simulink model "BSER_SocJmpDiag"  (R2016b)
settings: Solver=FixedStepDiscrete  StartTime=0.0  StopTime=10.0  FixedStep=0.02  RelTol=1e-3  EnableMultiTasking=on
undefined symbols (not defined in the file or in its folder): BSER_bSocJmpDiagSlct_CW, BSER_rBattSocValJmpFault_C, BSER_tiBattSocValJmpDiag_C, BSER_tiBattSocValJmpFault_C, BSER_tiSocValJmpErr_C, BSER_tiSocValJmpOk_C
libraries: simulink x6

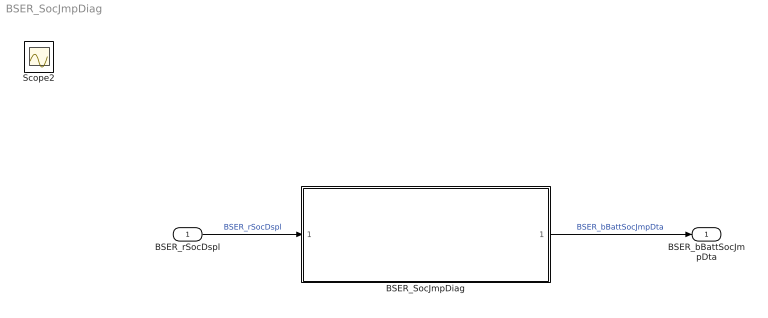
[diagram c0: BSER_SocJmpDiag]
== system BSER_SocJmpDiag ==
  BSER_rSocDspl : Inport
  BSER_SocJmpDiag : Subsystem
  BSER_bBattSocJmpDta : Outport
  Scope2 : Scope
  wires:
  BSER_rSocDspl/1 -> BSER_SocJmpDiag/1(BSER_rSocDspl)  "BSER_rSocDspl"
  BSER_SocJmpDiag/1(BSER_bBattSocJmpDta) -> BSER_bBattSocJmpDta/1  "BSER_bBattSocJmpDta"

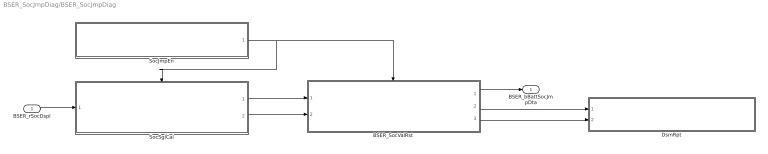
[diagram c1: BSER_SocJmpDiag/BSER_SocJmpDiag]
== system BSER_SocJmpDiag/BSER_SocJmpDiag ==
  BSER_rSocDspl : Inport
  BSER_SocValRst : Subsystem
  DsmRpt : Subsystem
  SocJmpEn : Subsystem
  SocSglCal : Subsystem
  BSER_bBattSocJmpDta : Outport
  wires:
  BSER_SocValRst/1(BSER_bBattSocJmpDta) -> BSER_bBattSocJmpDta/1
  SocJmpEn/1(BSER_bBattSocJmpEn) -> BSER_SocValRst/Enable, SocSglCal/Enable
  BSER_rSocDspl/1 -> SocSglCal/1(BSER_rSocDspl)
  SocSglCal/1(BSER_rSocDsplCont) -> BSER_SocValRst/1(BSER_rSocDsplCont)
  SocSglCal/2(BSER_rSocDsplPer) -> BSER_SocValRst/2(BSER_rSocDsplPer)
  BSER_SocValRst/2(BSER_bBattSocJmpFaultDet) -> DsmRpt/1(BSER_bBattSocJmpFaultDet)
  BSER_SocValRst/3(BSER_bBattSocJmpFaultHeal) -> DsmRpt/2(BSER_bBattSocJmpFaultHeal)

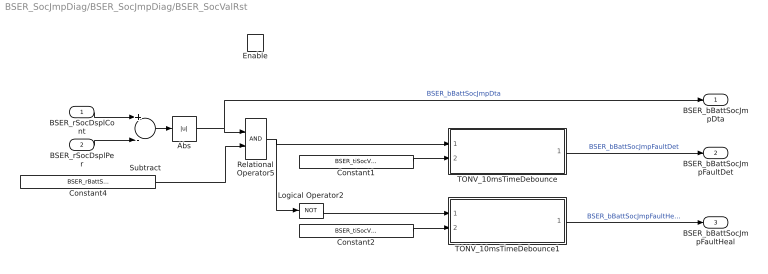
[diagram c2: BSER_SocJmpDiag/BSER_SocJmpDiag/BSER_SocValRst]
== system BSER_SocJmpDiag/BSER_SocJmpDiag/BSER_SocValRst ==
  BSER_rSocDsplCont : Inport
  BSER_rSocDsplPer : Inport  Port=2
  Enable : EnablePort  StatesWhenEnabling=reset
  Abs : Abs
  Constant1 : Constant  Value=BSER_tiSocValJmpErr_C
  Constant2 : Constant  Value=BSER_tiSocValJmpOk_C
  Constant4 : Constant  Value=BSER_rBattSocValJmpFault_C
  Logical Operator2 : Logic  Operator=NOT  AllPortsSameDT=off  OutDataTypeStr=boolean
  Relational Operator5 : RelationalOperator  OutDataTypeStr=boolean  RndMeth=Simplest
  Subtract : Sum  Inputs=+-  OutDataTypeStr=single
  TONV_10msTimeDebounce : Subsystem  TreatAsAtomicUnit=on  RTWFcnName=TONV_10msTimeDebounce  RTWFileName=SrvLib
  TONV_10msTimeDebounce1 : Subsystem  TreatAsAtomicUnit=on  RTWFcnName=TONV_10msTimeDebounce  RTWFileName=SrvLib
  BSER_bBattSocJmpDta : Outport  InitialOutput=[0]
  BSER_bBattSocJmpFaultDet : Outport  Port=2  InitialOutput=[0]
  BSER_bBattSocJmpFaultHeal : Outport  Port=3  InitialOutput=[0]
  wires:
  BSER_rSocDsplCont/1 -> Subtract/1
  Constant2/1 -> TONV_10msTimeDebounce1/2(T)
  Logical Operator2/1 -> TONV_10msTimeDebounce1/1(u)
  TONV_10msTimeDebounce1/1(y) -> BSER_bBattSocJmpFaultHeal/1  "BSER_bBattSocJmpFaultHeal"
  Constant1/1 -> TONV_10msTimeDebounce/2(T)
  TONV_10msTimeDebounce/1(y) -> BSER_bBattSocJmpFaultDet/1  "BSER_bBattSocJmpFaultDet"
  Constant4/1 -> Relational Operator5/2
  Subtract/1 -> Abs/1
  Abs/1 -> Relational Operator5/1, BSER_bBattSocJmpDta/1  "BSER_bBattSocJmpDta"
  Relational Operator5/1 -> Logical Operator2/1, TONV_10msTimeDebounce/1(u)
  BSER_rSocDsplPer/1 -> Subtract/2

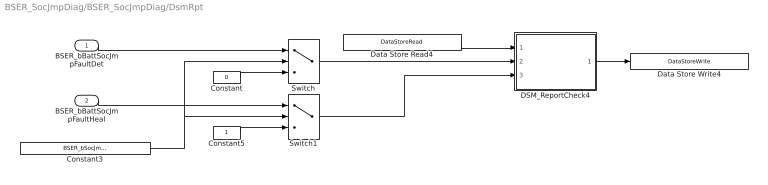
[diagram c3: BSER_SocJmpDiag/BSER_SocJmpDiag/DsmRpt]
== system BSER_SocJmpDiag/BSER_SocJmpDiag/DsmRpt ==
  BSER_bBattSocJmpFaultDet : Inport
  BSER_bBattSocJmpFaultHeal : Inport  Port=2
  Constant : Constant  Value=0  OutDataTypeStr=boolean
  Constant3 : Constant  Value=BSER_bSocJmpDiagSlct_CW
  Constant5 : Constant  OutDataTypeStr=boolean
  DSM_ReportCheck4 : Subsystem  TreatAsAtomicUnit=on  RTWFcnName=DSM_ReportCheck  RTWFileName=SrvLib
  Data Store Read4 : DataStoreRead  DataStoreName=DFC_SocValJmp
  Data Store Write4 : DataStoreWrite  DataStoreName=DFC_SocValJmp
  Switch : Switch  Criteria=u2 > Threshold
  Switch1 : Switch  Criteria=u2 > Threshold
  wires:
  DSM_ReportCheck4/1(Dfc_id) -> Data Store Write4/1
  Data Store Read4/1 -> DSM_ReportCheck4/1(Dfc_id_nv)
  Switch1/1 -> DSM_ReportCheck4/3(Heal)
  BSER_bBattSocJmpFaultDet/1 -> Switch/1
  BSER_bBattSocJmpFaultHeal/1 -> Switch1/1
  Constant/1 -> Switch/3
  Constant5/1 -> Switch1/3
  Constant3/1 -> Switch1/2, Switch/2
  Switch/1 -> DSM_ReportCheck4/2(Err)

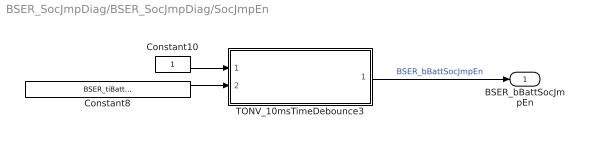
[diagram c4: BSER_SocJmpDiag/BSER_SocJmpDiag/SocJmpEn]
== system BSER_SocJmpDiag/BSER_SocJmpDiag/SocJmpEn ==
  Constant10 : Constant  OutDataTypeStr=boolean
  Constant8 : Constant  Value=BSER_tiBattSocValJmpDiag_C
  TONV_10msTimeDebounce3 : Subsystem  TreatAsAtomicUnit=on  RTWFcnName=TONV_10msTimeDebounce  RTWFileName=SrvLib
  BSER_bBattSocJmpEn : Outport
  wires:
  Constant8/1 -> TONV_10msTimeDebounce3/2(T)
  Constant10/1 -> TONV_10msTimeDebounce3/1(u)
  TONV_10msTimeDebounce3/1(y) -> BSER_bBattSocJmpEn/1  "BSER_bBattSocJmpEn"

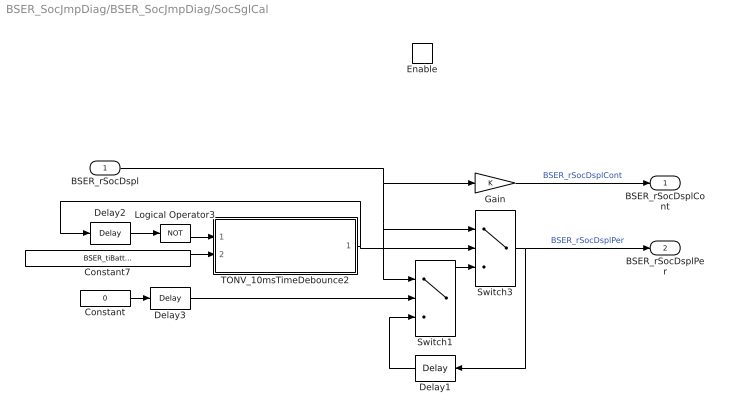
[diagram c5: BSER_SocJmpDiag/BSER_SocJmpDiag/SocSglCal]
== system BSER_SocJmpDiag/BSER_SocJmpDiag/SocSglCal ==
  BSER_rSocDspl : Inport
  Enable : EnablePort  StatesWhenEnabling=reset
  Constant : Constant  Value=0  OutDataTypeStr=uint8
  Constant7 : Constant  Value=BSER_tiBattSocValJmpFault_C
  Delay1 : Delay  DelayLength=1  InitialCondition=1
  Delay2 : Delay  DelayLength=1  InitialCondition=1
  Delay3 : Delay  DelayLength=1  InitialCondition=1
  Gain : Gain
  Logical Operator3 : Logic  Operator=NOT  AllPortsSameDT=off  OutDataTypeStr=boolean
  Switch1 : Switch  Criteria=u2 > Threshold
  Switch3 : Switch  Criteria=u2 > Threshold
  TONV_10msTimeDebounce2 : Subsystem  TreatAsAtomicUnit=on  RTWFcnName=TONV_10msTimeDebounce  RTWFileName=SrvLib
  BSER_rSocDsplCont : Outport
  BSER_rSocDsplPer : Outport  Port=2
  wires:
  Constant7/1 -> TONV_10msTimeDebounce2/2(T)
  Delay2/1 -> Logical Operator3/1
  Logical Operator3/1 -> TONV_10msTimeDebounce2/1(u)
  TONV_10msTimeDebounce2/1(y) -> Switch3/2, Delay2/1
  BSER_rSocDspl/1 -> Switch1/1, Switch3/1, Gain/1
  Switch3/1 -> BSER_rSocDsplPer/1, Delay1/1  "BSER_rSocDsplPer"
  Gain/1 -> BSER_rSocDsplCont/1  "BSER_rSocDsplCont"
  Constant/1 -> Delay3/1
  Delay3/1 -> Switch1/2
  Delay1/1 -> Switch1/3
  Switch1/1 -> Switch3/3

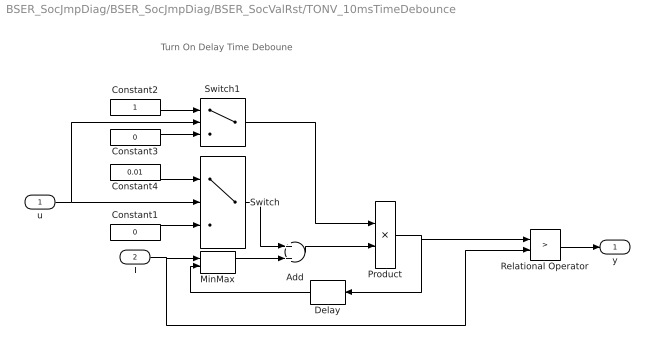
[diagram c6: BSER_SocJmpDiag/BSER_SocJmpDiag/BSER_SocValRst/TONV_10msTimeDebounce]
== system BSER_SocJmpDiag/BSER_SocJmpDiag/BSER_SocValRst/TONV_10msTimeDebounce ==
  note: Turn On Delay Time Deboune
  u : Inport
  T : Inport  Port=2
  Add : Sum
  Constant1 : Constant  Value=0  OutDataTypeStr=single
  Constant2 : Constant  OutDataTypeStr=uint8
  Constant3 : Constant  Value=0  OutDataTypeStr=uint8
  Constant4 : Constant  Value=0.01  OutDataTypeStr=single
  Delay : Delay  DelayLength=1  InitialCondition=0
  MinMax : MinMax  Inputs=2
  Product : Product  OutMin=[0]  OutMax=[65535]  OutDataTypeStr=single
  Relational Operator : RelationalOperator  Operator=>  OutDataTypeStr=boolean  RndMeth=Simplest
  Switch : Switch  Criteria=u2 ~= 0
  Switch1 : Switch  Criteria=u2 ~= 0
  y : Outport
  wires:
  MinMax/1 -> Add/2
  T/1 -> Relational Operator/2, MinMax/1
  Relational Operator/1 -> y/1
  Delay/1 -> MinMax/2
  Switch/1 -> Add/1
  Product/1 -> Delay/1, Relational Operator/1
  Add/1 -> Product/2
  Constant1/1 -> Switch/3
  Constant4/1 -> Switch/1
  u/1 -> Switch/2, Switch1/2
  Constant2/1 -> Switch1/1
  Constant3/1 -> Switch1/3
  Switch1/1 -> Product/1

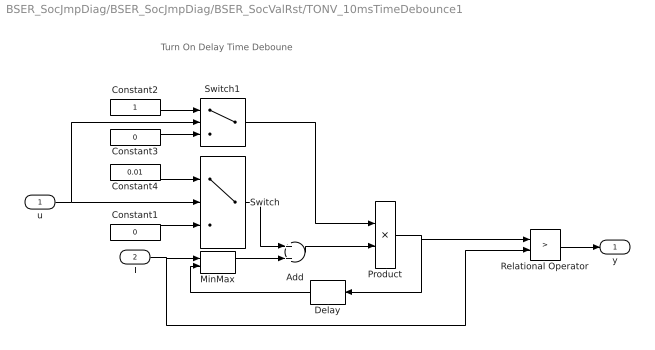
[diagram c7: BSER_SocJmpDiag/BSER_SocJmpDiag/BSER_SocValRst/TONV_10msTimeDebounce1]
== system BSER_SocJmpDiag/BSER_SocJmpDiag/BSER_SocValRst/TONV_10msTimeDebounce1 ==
  note: Turn On Delay Time Deboune
  u : Inport
  T : Inport  Port=2
  Add : Sum
  Constant1 : Constant  Value=0  OutDataTypeStr=single
  Constant2 : Constant  OutDataTypeStr=uint8
  Constant3 : Constant  Value=0  OutDataTypeStr=uint8
  Constant4 : Constant  Value=0.01  OutDataTypeStr=single
  Delay : Delay  DelayLength=1  InitialCondition=0
  MinMax : MinMax  Inputs=2
  Product : Product  OutMin=[0]  OutMax=[65535]  OutDataTypeStr=single
  Relational Operator : RelationalOperator  Operator=>  OutDataTypeStr=boolean  RndMeth=Simplest
  Switch : Switch  Criteria=u2 ~= 0
  Switch1 : Switch  Criteria=u2 ~= 0
  y : Outport
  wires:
  Switch1/1 -> Product/1
  Constant3/1 -> Switch1/3
  Constant2/1 -> Switch1/1
  u/1 -> Switch1/2, Switch/2
  Constant4/1 -> Switch/1
  Constant1/1 -> Switch/3
  Add/1 -> Product/2
  Product/1 -> Relational Operator/1, Delay/1
  Switch/1 -> Add/1
  Delay/1 -> MinMax/2
  Relational Operator/1 -> y/1
  T/1 -> MinMax/1, Relational Operator/2
  MinMax/1 -> Add/2

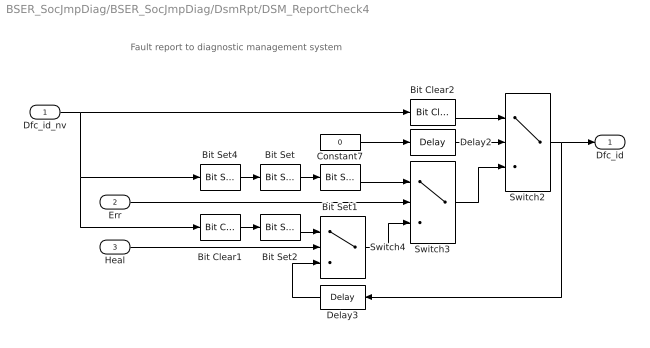
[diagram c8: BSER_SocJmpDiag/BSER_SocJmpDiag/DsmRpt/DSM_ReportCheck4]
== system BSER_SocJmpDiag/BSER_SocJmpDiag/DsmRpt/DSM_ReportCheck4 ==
  note: Fault report to diagnostic management system
  Dfc_id_nv : Inport  OutDataTypeStr=uint8
  Err : Inport  Port=2
  Heal : Inport  Port=3
  Bit Clear1 : simulink/Logic and Bit Operations/Bit Clear  iBit=4
  Bit Clear2 : simulink/Logic and Bit Operations/Bit Clear  iBit=3
  Bit Set : simulink/Logic and Bit Operations/Bit Set  iBit=4
  Bit Set1 : simulink/Logic and Bit Operations/Bit Set  iBit=3
  Bit Set2 : simulink/Logic and Bit Operations/Bit Set  iBit=3
  Bit Set4 : simulink/Logic and Bit Operations/Bit Set  iBit=7
  Constant7 : Constant  Value=0  OutDataTypeStr=boolean
  Delay2 : Delay  DelayLength=1  InitialCondition=1
  Delay3 : Delay  DelayLength=1  InitialCondition=0
  Switch2 : Switch  Criteria=u2 ~= 0
  Switch3 : Switch  Criteria=u2 ~= 0
  Switch4 : Switch  Criteria=u2 ~= 0
  Dfc_id : Outport  OutDataTypeStr=uint8
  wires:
  Dfc_id_nv/1 -> Bit Clear2/1, Bit Set4/1, Bit Clear1/1
  Bit Set4/1 -> Bit Set/1
  Constant7/1 -> Delay2/1
  Delay2/1 -> Switch2/2
  Switch3/1 -> Switch2/3
  Bit Clear2/1 -> Switch2/1
  Switch2/1 -> Delay3/1, Dfc_id/1
  Bit Set1/1 -> Switch3/1
  Bit Set/1 -> Bit Set1/1
  Switch4/1 -> Switch3/3
  Err/1 -> Switch3/2
  Bit Set2/1 -> Switch4/1
  Bit Clear1/1 -> Bit Set2/1
  Delay3/1 -> Switch4/3
  Heal/1 -> Switch4/2

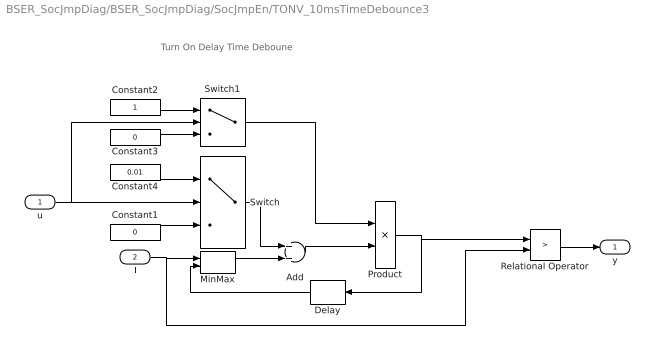
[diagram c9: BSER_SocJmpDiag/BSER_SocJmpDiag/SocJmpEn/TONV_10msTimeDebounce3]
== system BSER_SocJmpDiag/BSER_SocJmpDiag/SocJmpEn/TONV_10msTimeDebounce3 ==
  note: Turn On Delay Time Deboune
  u : Inport
  T : Inport  Port=2
  Add : Sum
  Constant1 : Constant  Value=0  OutDataTypeStr=single
  Constant2 : Constant  OutDataTypeStr=uint8
  Constant3 : Constant  Value=0  OutDataTypeStr=uint8
  Constant4 : Constant  Value=0.01  OutDataTypeStr=single
  Delay : Delay  DelayLength=1  InitialCondition=0
  MinMax : MinMax  Inputs=2
  Product : Product  OutMin=[0]  OutMax=[65535]  OutDataTypeStr=single
  Relational Operator : RelationalOperator  Operator=>  OutDataTypeStr=boolean  RndMeth=Simplest
  Switch : Switch  Criteria=u2 ~= 0
  Switch1 : Switch  Criteria=u2 ~= 0
  y : Outport
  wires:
  Switch1/1 -> Product/1
  Constant3/1 -> Switch1/3
  Constant2/1 -> Switch1/1
  u/1 -> Switch1/2, Switch/2
  Constant4/1 -> Switch/1
  Constant1/1 -> Switch/3
  Add/1 -> Product/2
  Product/1 -> Relational Operator/1, Delay/1
  Switch/1 -> Add/1
  Delay/1 -> MinMax/2
  Relational Operator/1 -> y/1
  T/1 -> MinMax/1, Relational Operator/2
  MinMax/1 -> Add/2

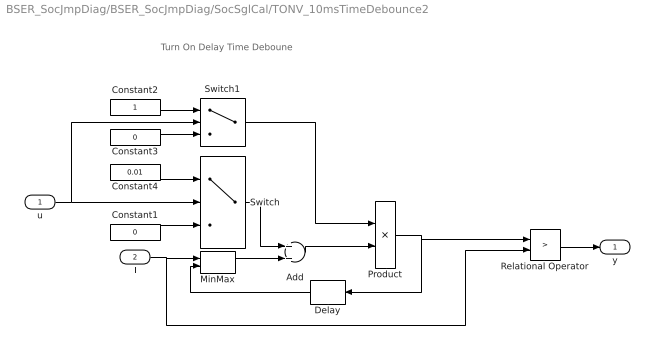
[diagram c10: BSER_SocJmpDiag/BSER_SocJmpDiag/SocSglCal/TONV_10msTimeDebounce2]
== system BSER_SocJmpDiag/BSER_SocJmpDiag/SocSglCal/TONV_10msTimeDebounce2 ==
  note: Turn On Delay Time Deboune
  u : Inport
  T : Inport  Port=2
  Add : Sum
  Constant1 : Constant  Value=0  OutDataTypeStr=single
  Constant2 : Constant  OutDataTypeStr=uint8
  Constant3 : Constant  Value=0  OutDataTypeStr=uint8
  Constant4 : Constant  Value=0.01  OutDataTypeStr=single
  Delay : Delay  DelayLength=1  InitialCondition=0
  MinMax : MinMax  Inputs=2
  Product : Product  OutMin=[0]  OutMax=[65535]  OutDataTypeStr=single
  Relational Operator : RelationalOperator  Operator=>  OutDataTypeStr=boolean  RndMeth=Simplest
  Switch : Switch  Criteria=u2 ~= 0
  Switch1 : Switch  Criteria=u2 ~= 0
  y : Outport
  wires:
  MinMax/1 -> Add/2
  T/1 -> Relational Operator/2, MinMax/1
  Relational Operator/1 -> y/1
  Delay/1 -> MinMax/2
  Switch/1 -> Add/1
  Product/1 -> Delay/1, Relational Operator/1
  Add/1 -> Product/2
  Constant1/1 -> Switch/3
  Constant4/1 -> Switch/1
  u/1 -> Switch/2, Switch1/2
  Constant2/1 -> Switch1/1
  Constant3/1 -> Switch1/3
  Switch1/1 -> Product/1
